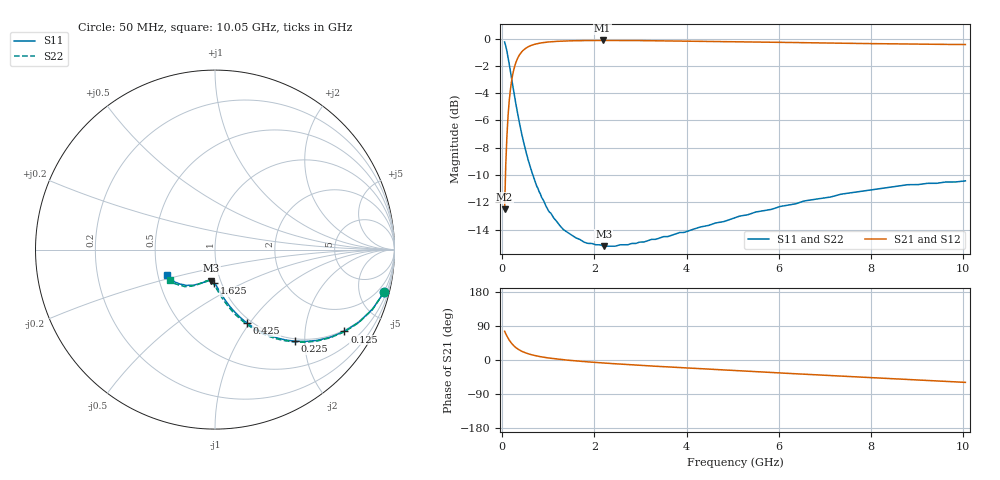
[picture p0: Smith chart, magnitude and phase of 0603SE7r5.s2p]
! AVX Thin Film Operation		Date: August 2001
! Description: Accu-P® Series, Thin Film, SMD, RF Capacitor
! Part Number: 06035J7R5BBT
! 50 MHz  -  10.05 GHz
! Serial Measurements
# mhz S db R 50
!	S11		S21		S12		S22
!	dB	Phase	dB	Phase	dB	Phase	dB	Phase
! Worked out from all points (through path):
!   401 points, 50 MHz to 10.05 GHz, reference 50 ohm
!   highest |S21| = -0.14 dB at 2.175 GHz (marker M1); lowest = -12.5 dB at 50 MHz (marker M2)
!   group delay of S21, straight-line fit = 21.8 ps
!   lowest |S11| = -15.2 dB at 2.2 GHz (marker M3), VSWR 1.42, Z = 45.3 - j16.1 ohm
!   |S11| at or under -10 dB: 664.6 MHz to end of sweep
!   |S22| runs from -15.2 to -0.3 dB; largest |S21 - S12| = 0
!   S11 on the Smith chart (normalised r, x): 50 MHz: 0.95, -7.97; 125 MHz: 0.95, -3.19; 225 MHz: 0.95, -1.79; 425 MHz: 0.95, -0.97; 1.625 GHz: 0.93, -0.36; 10.05 GHz: 0.56, -0.18
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50  -0.25 -14.1  -12.50 75.8  -12.50 75.8  -0.25 -14.2
75  -0.55 -20.6  -9.26 69.3  -9.26 69.3  -0.55 -20.8
125  -1.38 -32.3  -5.65 57.5  -5.65 57.5  -1.38 -32.6
175  -2.37 -41.6  -3.77 48.1  -3.77 48.1  -2.37 -42.1
225  -3.40 -49.0  -2.65 40.7  -2.65 40.7  -3.40 -49.5
275  -4.41 -54.9  -1.96 34.7  -1.96 34.7  -4.41 -55.6
325  -5.36 -59.6  -1.50 30.0  -1.50 30.0  -5.36 -60.4
425  -7.04 -66.5  -0.96 22.9  -0.96 22.9  -7.04 -67.5
525  -8.44 -71.3  -0.68 18.0  -0.68 18.0  -8.43 -72.6
650  -9.86 -75.8  -0.48 13.4  -0.48 13.4  -9.86 -77.2
975  -12.43 -83.1  -0.26 5.9  -0.26 5.9  -12.43 -85.0
1300  -13.89 -87.7  -0.19 1.0  -0.19 1.0  -13.89 -89.9
1625  -14.63 -91.3  -0.16 -2.6  -0.16 -2.6  -14.63 -93.6
1725  -14.80 -92.3  -0.15 -3.7  -0.15 -3.7  -14.80 -94.6
2175  -15.17 -96.5  -0.14 -7.8  -0.14 -7.8  -15.10 -98.6
2200  -15.20 -96.7  -0.14 -8.0  -0.14 -8.0  -15.10 -98.8
2700  -15.10 -100.8  -0.15 -11.9  -0.15 -11.9  -15.10 -102.8
3400  -14.62 -106.0  -0.16 -17.0  -0.16 -17.0  -14.62 -107.0
5050  -13.12 -118.4  -0.23 -28.0  -0.23 -28.0  -13.12 -117.4
6725  -11.80 -129.0  -0.31 -38.5  -0.31 -38.5  -11.80 -127.0
8400  -10.89 -140.2  -0.39 -49.0  -0.39 -49.0  -10.89 -137.1
10050  -10.42 -151.6  -0.44 -59.0  -0.44 -59.0  -10.40 -145.8
